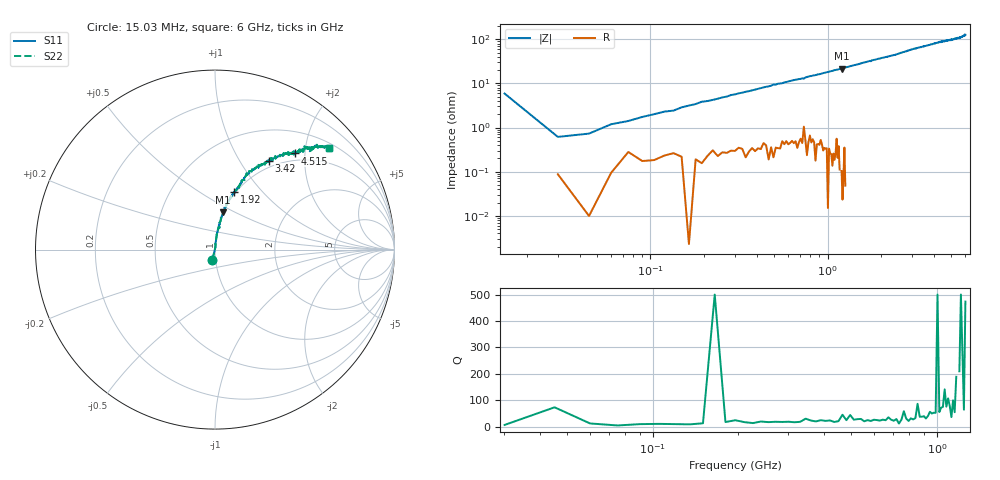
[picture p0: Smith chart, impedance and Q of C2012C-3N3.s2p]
!	Network	Analyzer	HP8753E.07.74:	Oct	30	2002	Serial	No.	JP38451487
!	Hewlett-Packard
!	7	Sep	2009	10:38:55
!	Frequency	S11	S21	S12	S22
#	HZ	S	RI	R	50
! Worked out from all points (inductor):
!   400 points, 15.03 MHz to 6 GHz, reference 50 ohm
!   read as one part in series: L = 2.92 nH near 45.03 MHz
!   highest Q = 189 at 1.2 GHz (marker M1), where L = 2.88 nH
!   S11 on the Smith chart (normalised r, x): 15.03 MHz: 0.96, -0.11; 1.92 GHz: 0.98, +0.71; 3.42 GHz: 0.91, +1.35; 4.515 GHz: 0.86, +1.80; 6 GHz: 0.61, +2.49
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1.502992e7  -0.015 -0.0572  1.02 0.0572  1.02 0.0572  -0.015 -0.0572
3.002985e7  0.000818 0.00606  0.999 -0.00606  0.999 -0.00606  0.000818 0.00606
4.502978e7  0.000304 0.00728  1 -0.00728  1 -0.00728  0.000304 0.00728
6.00297e7  0.00116 0.0118  0.999 -0.0118  0.999 -0.0118  0.00116 0.0118
1.200294e8  0.00266 0.0227  0.997 -0.0227  0.997 -0.0227  0.00266 0.0227
1.95029e8  0.00303 0.0382  0.997 -0.0382  0.997 -0.0382  0.00303 0.0382
2.850286e8  0.00581 0.0539  0.994 -0.0539  0.994 -0.0539  0.00581 0.0539
4.950275e8  0.0106 0.0927  0.989 -0.0927  0.989 -0.0927  0.0106 0.0927
1.020025e9  0.0356 0.177  0.964 -0.177  0.964 -0.177  0.0356 0.177
1.200024e9  0.0459 0.207  0.954 -0.207  0.954 -0.207  0.0459 0.207
1.92002e9  0.107 0.321  0.893 -0.321  0.893 -0.321  0.107 0.321
2.01002e9  0.118 0.331  0.882 -0.331  0.882 -0.331  0.118 0.331
3.015015e9  0.243 0.472  0.757 -0.472  0.757 -0.472  0.243 0.472
3.420013e9  0.301 0.495  0.699 -0.495  0.699 -0.495  0.301 0.495
4.00501e9  0.383 0.538  0.617 -0.538  0.617 -0.538  0.383 0.538
4.515007e9  0.445 0.536  0.555 -0.536  0.555 -0.536  0.445 0.536
5.010005e9  0.484 0.554  0.516 -0.554  0.516 -0.554  0.484 0.554
5.535002e9  0.528 0.548  0.472 -0.548  0.472 -0.548  0.528 0.548
5.565002e9  0.56 0.58  0.44 -0.58  0.44 -0.58  0.56 0.58
5.595002e9  0.536 0.57  0.464 -0.57  0.464 -0.57  0.536 0.57
5.625002e9  0.57 0.575  0.43 -0.575  0.43 -0.575  0.57 0.575
6e9  0.633 0.566  0.367 -0.566  0.367 -0.566  0.633 0.566
